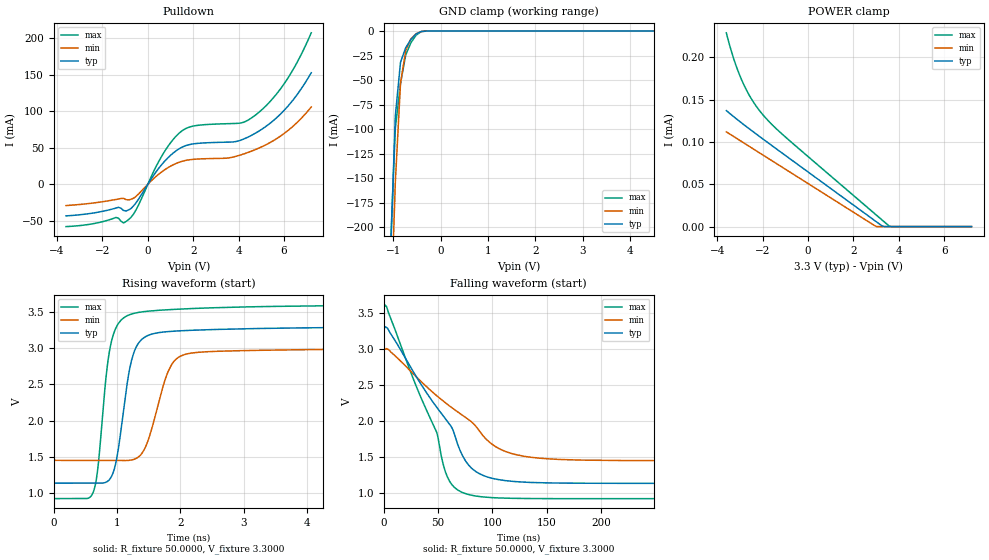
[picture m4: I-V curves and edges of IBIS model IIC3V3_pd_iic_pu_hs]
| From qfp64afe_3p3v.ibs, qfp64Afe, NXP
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[Model] IIC3V3_pd_iic_pu_hs
|   Model IIC3V3_pd_iic_pu_hs
| This model was characterised for following simulation conditions:
| External (pad) voltage:
|   - Typ: 3.3V,   - Min: 3.0V,   - Max: 3.6V
| Library cells for typ/min/max conditions are connected as defined below:
|  IO - External Pad
|  A - Core Input
|  EN - Output Buffer Enable
|  BOOST - vdde
|  ECS - vdd
|  EGP - gnd
|  ENZI - vdd
|  EPD - vdd
|  EPUN - vdd
|  SSEL - vdd
|  ZI - NC
|  ZIF - NC
|  gnd - gnd
|  gnde - gnde
|  vdd - vdd
|  vdde - vdde
| All other pins connected to ground
Model_type I/O_open_drain
Polarity   Non-Inverting
Enable   Active-Low
Vinl =   0.9900V
Vinh =   2.3100V
Vmeas =  1.6500V
Cref =   0.0F
Rref =   1.0000k
Vref =   3.3000V
C_comp   3.5907pF   3.4406pF   3.7387pF
|C_comp_pullup   0.9138pF   0.8999pF   0.9173pF
|C_comp_pulldown   2.3268pF   2.4803pF   2.1806pF
[Model Spec]
| variable   typ   min   max
Vinh   0.9900V   0.9000V   1.0800V
Vinl   2.3100V   2.1000V   2.5200V
Vmeas   1.6500V   1.5000V   1.8000V
Vref   3.3000V   3.0000V   3.6000V
Cref   0.0F   0.0F   0.0F
Rref   1.0000k   1.0000k   1.0000k
[Temperature Range]   25.0000   0.1250k   -40.0000
[Voltage Range]   3.3000V   3.0000V   3.6000V
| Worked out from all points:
|   slope of the pulldown table from 0 to 0.495 V, typ, clamps not added: 22 ohm
|   GND clamp passes 1 mA (typ) near -0.43 V on its own axis
|   rising waveform, R_fixture 50.0000, V_fixture 3.3000: 20-80 % time 227ps typ, 309ps min, 192ps max; typ from 1.14 V to 3.3 V
|   falling waveform, R_fixture 50.0000, V_fixture 3.3000: 20-80 % time 50.8ns typ, 68.6ns min, 38.5ns max; typ from 3.3 V to 1.14 V
[Pulldown]
|Voltage   I(typ)   I(min)   I(max)
-3.6V     -43.22mA   -29.09mA   -57.9mA
-1.29V    -31.46mA   -20.15mA   -46.47mA
-1.07V    -35.79mA   -19.19mA   -52.9mA
-850mV    -35.14mA   -21.36mA   -48.43mA
-520mV    -25.35mA   -16.52mA   -35.11mA
580mV     25.81mA    16.3mA     36.8mA
1.24V     45.79mA    28.53mA    65.82mA
1.9V      54.89mA    33.9mA     79.08mA
4.1V      60.55mA    40.38mA    84.05mA
4.76V     70.44mA    47.87mA    95.32mA
6.08V     103.9mA    71.39mA    141.2mA
7.2V      152.9mA    106mA      207.6mA
[GND_clamp]
|Voltage   I(typ)   I(min)   I(max)
-3.6V     -5.602A    -5.487A    -5.717A
-1.07V    -242mA     -316.8mA   -230.5mA
-960mV    -86.76mA   -154.7mA   -99.49mA
-850mV    -31.82mA   -53.09mA   -53.51mA
-740mV    -16.97mA   -19.87mA   -24.44mA
-630mV    -8.597mA   -7.926mA   -11.89mA
-520mV    -3.004mA   -2.733mA   -4.196mA
-410mV    -439.7uA   -501.8uA   -589.4uA
7.2V      0A         0A         0A
[POWER_clamp]
|Voltage   I(typ)   I(min)   I(max)
-3.6V     137uA      111.9uA    228.9uA
-3.47V    134.1uA    109.7uA    215.6uA
-3.25V    129.3uA    106uA      196.2uA
-2.92V    122.3uA    100.4uA    172.9uA
-2.48V    113.3uA    92.88uA    150.2uA
-2.04V    104.5uA    85.42uA    133.7uA
-1.16V    87.2uA     70.51uA    109.7uA
2.91V     7.626uA    1.527uA    15.86uA
3.02V     5.475uA    0A         13.33uA
3.24V     1.173uA    0A         8.273uA
3.57V     0A         0A         687.1nA
7.2V      0A         0A         0A
[Ramp]
| variable   typ   min   max
dV/dt_r  1.2983/0.2270n   0.9293/0.3088n   1.6062/0.1924n
dV/dt_f  1.2983/50.7687n   0.9293/68.6294n   1.6062/38.4596n
R_load = 50.0000
[Rising Waveform]
R_fixture= 50.0000
V_fixture= 3.3000
V_fixture_min= 3.0000
V_fixture_max= 3.6000
|time   V(typ)   V(min)   V(max)
0s        1.135V     1.45V      921.3mV
623.8ps   1.134V     1.45V      1.013V
886.4ps   1.192V     1.45V      2.995V
994.5ps   1.48V      1.449V     3.305V
1.153ns   2.479V     1.448V     3.447V
1.389ns   3.121V     1.544V     3.502V
1.808ns   3.23V      2.683V     3.532V
2.031ns   3.242V     2.902V     3.542V
5.392ns   3.291V     2.989V     3.591V
1us       3.299V     2.999V     3.598V
[Falling Waveform]
R_fixture= 50.0000
V_fixture= 3.3000
V_fixture_min= 3.0000
V_fixture_max= 3.6000
|time   V(typ)   V(min)   V(max)
0s        3.299V     2.999V     3.598V
2.486ns   3.299V     3.008V     3.588V
48.47ns   2.195V     2.355V     1.849V
54.55ns   2.074V     2.279V     1.404V
59.69ns   1.974V     2.218V     1.185V
72ns      1.531V     2.085V     1.01V
83.39ns   1.313V     1.951V     961.5mV
112.3ns   1.172V     1.576V     928.6mV
164.5ns   1.138V     1.465V     921.8mV
1us       1.135V     1.45V      921.3mV
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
